FUNCTION_BLOCK Run_Blend_DUT

VAR_IN_OUT
    SD_SMD_IO: DUT_AMCI_Stepper;
END_VAR	

VAR_INPUT
	FB_0_CW_1_CCW: BOOL;
		
END_VAR

VAR_OUTPUT
	Enable: BOOL :=FALSE;
	Error: BOOL :=TRUE;
END_VAR

VAR	
	I_Command_Word_1: UINT;
		
END_VAR
VAR // added by the converter: edge detectors and wires of the graphical bodies
    _w1, _w2 : BOOL;
END_VAR

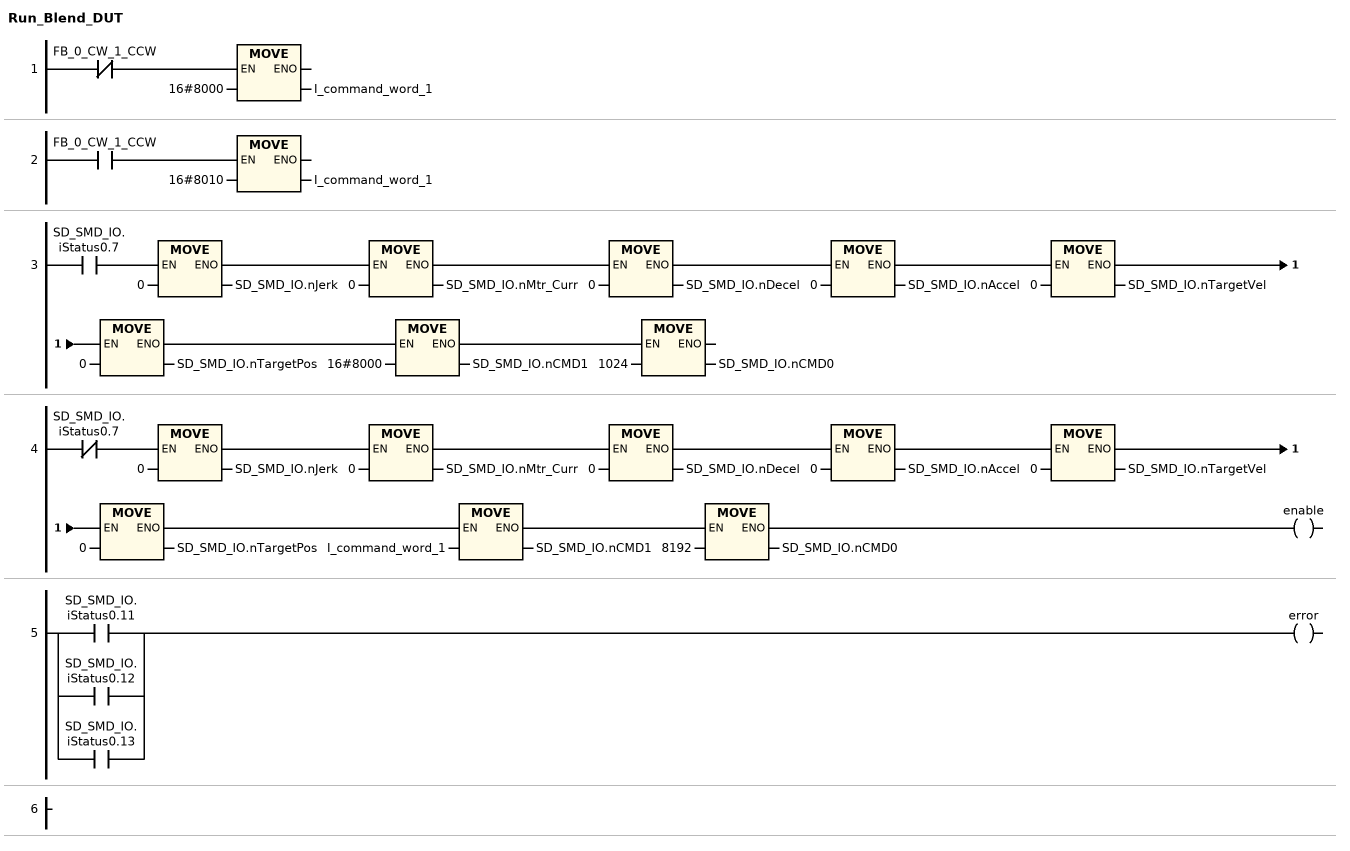
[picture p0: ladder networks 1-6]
// NETWORK 1
IF NOT FB_0_CW_1_CCW THEN I_command_word_1 := 16#8000; END_IF

// NETWORK 2
IF FB_0_CW_1_CCW THEN I_command_word_1 := 16#8010; END_IF

// NETWORK 3
_w1 := SD_SMD_IO.iStatus0.7;
IF _w1 THEN SD_SMD_IO.nJerk := 0; END_IF
IF _w1 THEN SD_SMD_IO.nMtr_Curr := 0; END_IF
IF _w1 THEN SD_SMD_IO.nDecel := 0; END_IF
IF _w1 THEN SD_SMD_IO.nAccel := 0; END_IF
IF _w1 THEN SD_SMD_IO.nTargetVel := 0; END_IF
IF _w1 THEN SD_SMD_IO.nTargetPos := 0; END_IF
IF _w1 THEN SD_SMD_IO.nCMD1 := 16#8000; END_IF
IF _w1 THEN SD_SMD_IO.nCMD0 := 1024; END_IF

// NETWORK 4
_w2 := NOT SD_SMD_IO.iStatus0.7;
IF _w2 THEN SD_SMD_IO.nJerk := 0; END_IF
IF _w2 THEN SD_SMD_IO.nMtr_Curr := 0; END_IF
IF _w2 THEN SD_SMD_IO.nDecel := 0; END_IF
IF _w2 THEN SD_SMD_IO.nAccel := 0; END_IF
IF _w2 THEN SD_SMD_IO.nTargetVel := 0; END_IF
IF _w2 THEN SD_SMD_IO.nTargetPos := 0; END_IF
IF _w2 THEN SD_SMD_IO.nCMD1 := I_command_word_1; END_IF
IF _w2 THEN SD_SMD_IO.nCMD0 := 8192; END_IF
enable := _w2;

// NETWORK 5
error := SD_SMD_IO.iStatus0.11 OR SD_SMD_IO.iStatus0.12 OR SD_SMD_IO.iStatus0.13;

// NETWORK 6

END_FUNCTION_BLOCK
